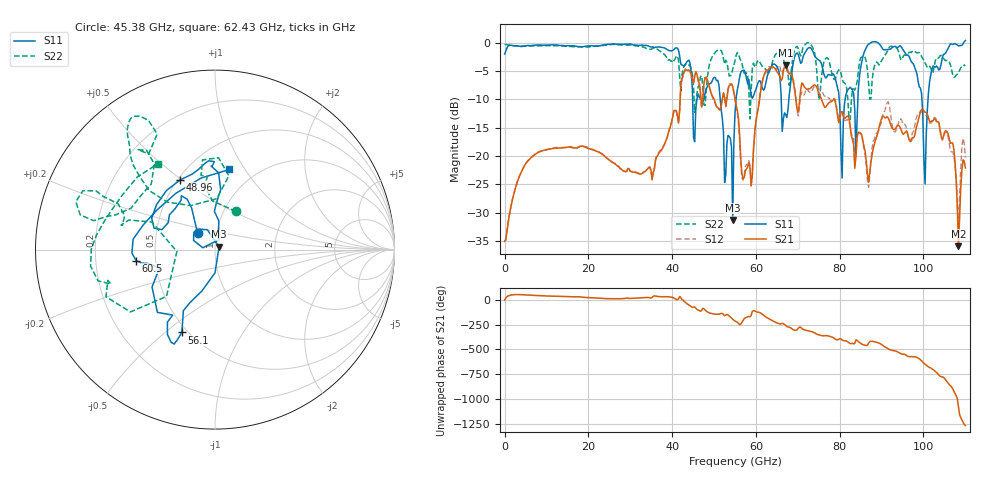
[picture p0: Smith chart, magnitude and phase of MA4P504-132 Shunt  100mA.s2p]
!Keysight Technologies,N5247B,US61255204,A.15.70.20
!Date: Friday, October 21, 2022 15:00:24
!Correction: S11(C  4-Port  )
!S31(C  4-Port  )
!S13(C  4-Port  )
!S33(C  4-Port  )
!S2P File: Measurements: S11, S31, S13, S33:
# Hz S  dB  R 50
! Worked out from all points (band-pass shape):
!   401 points, 10 MHz to 110 GHz, reference 50 ohm
!   highest |S21| = -3.95 dB at 67.1 GHz (marker M1); lowest = -35.9 dB at 108.4 GHz (marker M2)
!   |S21| within 3 dB of the highest: 42.14 GHz to 45.03 GHz (2.883 GHz wide, 6.61 % of centre); 61.52 GHz to 68.94 GHz (7.424 GHz wide, 11.4 % of centre)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
!   lowest |S11| = -31.3 dB at 54.46 GHz (marker M3), VSWR 1.06, Z = 52.3 + j1.62 ohm
!   |S11| at or under -10 dB: 51.49 GHz to 55.25 GHz (3.756 GHz wide, 7.04 % of centre); 66.04 GHz to 67.86 GHz (1.819 GHz wide, 2.72 % of centre); 79.89 GHz to 81.3 GHz (1.41 GHz wide, 1.75 % of centre)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
!   |S22| runs from -13.5 to 0.0 dB; largest |S21 - S12| = 0.24
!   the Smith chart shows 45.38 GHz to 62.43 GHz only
!   S11 on the Smith chart (normalised r, x): 45.38 GHz: 0.81, +0.15; 48.96 GHz: 0.52, +0.49; 56.1 GHz: 0.47, -0.57; 60.5 GHz: 0.39, -0.06; 62.43 GHz: 0.76, +0.85
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1e7  -1.97 -180.0  -35.05 -3.5  -35.02 -3.5  -0.28 179.8
1.843332e10  -0.71 118.1  -18.23 28.0  -18.25 28.1  -0.69 124.8
3.685665e10  -0.73 115.7  -19.46 33.1  -19.29 33.1  -1.32 122.5
4.373102e10  -3.19 18.4  -4.88 -44.4  -4.72 -42.3  -4.02 82.1
4.538088e10  -17.47 136.6  -5.93 -72.3  -5.85 -71.5  -12.26 61.0
4.895555e10  -7.25 116.3  -7.97 -133.1  -7.92 -131.2  -3.66 134.0
5.445505e10  -31.29 34.5  -7.70 165.2  -7.78 164.5  -4.63 160.7
5.5005e10  -12.32 -107.6  -9.89 146.9  -10.11 145.2  -3.15 166.6
5.61049e10  -6.07 -111.8  -16.23 111.6  -17.14 115.3  -2.64 153.7
6.05045e10  -7.06 -172.0  -11.79 -125.1  -11.43 -120.1  -3.11 -172.4
6.242932e10  -6.87 79.8  -4.91 -174.1  -5.16 -167.7  -4.81 123.5
6.462912e10  -3.83 17.0  -4.57 134.4  -4.72 155.8  -2.10 63.3
6.71039e10  -12.68 -39.1  -3.95 102.2  -3.63 102.7  -4.28 45.8
7.342832e10  -1.25 139.1  -7.72 38.2  -8.42 36.6  -0.66 108.9
8.112762e10  -10.85 -28.3  -13.35 -51.3  -13.67 -52.0  -7.08 -125.5
8.525225e10  -3.40 39.6  -16.24 -85.4  -16.35 -84.0  -2.53 -22.7
9.185165e10  -1.15 91.1  -13.74 -139.8  -11.09 -133.7  -0.77 84.1
9.872602e10  -6.89 150.4  -13.70 133.5  -12.47 133.1  -1.72 177.0
1.003759e11  -24.92 -11.6  -12.24 71.9  -12.68 73.9  -3.57 -156.2
1.036756e11  -4.82 -33.8  -14.14 -37.8  -14.01 -34.3  -2.60 -89.6
1.083502e11  -0.54 22.2  -35.91 5.1  -33.40 10.2  -5.18 -5.4
1.1e11  0.42 54.5  -22.11 174.0  -20.27 176.0  -4.06 16.4
